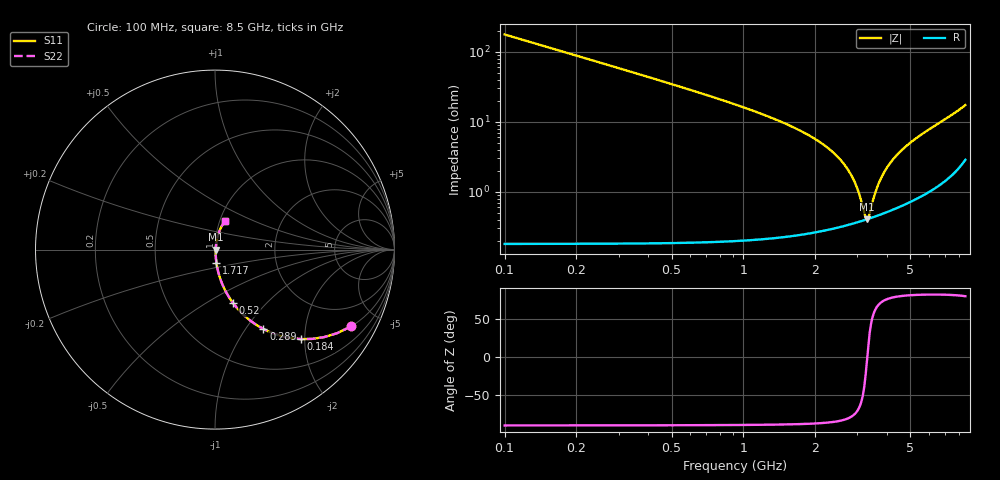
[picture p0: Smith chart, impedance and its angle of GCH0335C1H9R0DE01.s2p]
!Murata Part Number: GCH0335C1H9R0DE01
!These Parameters are Measured in Series Mode Connection
!Data Generated on Mar 13, 2026
!  o--ll--o
!Port1  Port2
!  o------o
!Operation Temp=25[degC], DC Bias Voltage=0[V]
!Freq. Start=100[MHz] Stop=9[GHz] 401[Steps]
# Hz S RI R 50
!Freq.(Hz) S11(Real) S11(Imag) S21(Real) S21(Imag) S12(Real) S12(Imag) S22(Real) S22(Imag)
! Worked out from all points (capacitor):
!   401 points, 100 MHz to 8.5 GHz, reference 50 ohm
!   read as one part in series: C = 9 pF near 142 MHz
!   lowest |Z| = 406 mohm at 3.292 GHz (marker M1)
!   series resonance near 3.299 GHz, so ESL is about 260 pH
!   S11 on the Smith chart (normalised r, x): 100 MHz: 1.00, -3.53; 184 MHz: 1.00, -1.92; 289 MHz: 1.00, -1.21; 520 MHz: 1.00, -0.66; 1.717 GHz: 1.00, -0.15; 8.5 GHz: 1.06, +0.34
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1e8  0.7572 -0.4283  0.2428 0.4283  0.2428 0.4283  0.7572 -0.4283
1.84e8  0.4787 -0.4986  0.5213 0.4986  0.5213 0.4986  0.4787 -0.4986
2.89e8  0.2701 -0.4425  0.7299 0.4425  0.7299 0.4425  0.2701 -0.4425
3.94e8  0.1648 -0.369  0.8352 0.369  0.8352 0.369  0.1648 -0.369
5.2e8  0.1005 -0.2979  0.8995 0.2979  0.8995 0.2979  0.1005 -0.2979
8.98e8  0.0341 -0.1761  0.9659 0.1761  0.9659 0.1761  0.0341 -0.1761
1.507e9  0.0109 -0.0922  0.9891 0.0922  0.9891 0.0922  0.0109 -0.0922
1.717e9  0.00806 -0.0749  0.9919 0.0749  0.9919 0.0749  0.00806 -0.0749
2.473e9  0.00406 -0.0316  0.9959 0.0316  0.9959 0.0316  0.00406 -0.0316
2.914e9  0.00373 -0.0136  0.9963 0.0136  0.9963 0.0136  0.00373 -0.0136
3.061e9  0.0038 -0.00818  0.9962 0.00818  0.9962 0.00818  0.0038 -0.00818
3.229e9  0.00396 -0.00234  0.996 0.00234  0.996 0.00234  0.00396 -0.00234
3.292e9  0.00404 -0.000226  0.996 0.000226  0.996 0.000226  0.00404 -0.000226
3.355e9  0.00413 0.00186  0.9959 -0.00186  0.9959 -0.00186  0.00413 0.00186
3.544e9  0.00446 0.00791  0.9955 -0.00791  0.9955 -0.00791  0.00446 0.00791
3.733e9  0.00487 0.0137  0.9951 -0.0137  0.9951 -0.0137  0.00487 0.0137
3.985e9  0.00554 0.0212  0.9945 -0.0212  0.9945 -0.0212  0.00554 0.0212
4.3e9  0.00656 0.0301  0.9934 -0.0301  0.9934 -0.0301  0.00656 0.0301
4.888e9  0.00899 0.046  0.991 -0.046  0.991 -0.046  0.00899 0.046
5.707e9  0.0136 0.0678  0.9864 -0.0678  0.9864 -0.0678  0.0136 0.0678
7.114e9  0.0266 0.1077  0.9734 -0.1077  0.9734 -0.1077  0.0266 0.1077
8.5e9  0.0541 0.1573  0.9459 -0.1573  0.9459 -0.1573  0.0541 0.1573
